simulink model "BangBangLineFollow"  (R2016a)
settings: Solver=FixedStepAuto  StartTime=0.0  StopTime=inf  RelTol=1e-3
libraries: miniQ x2

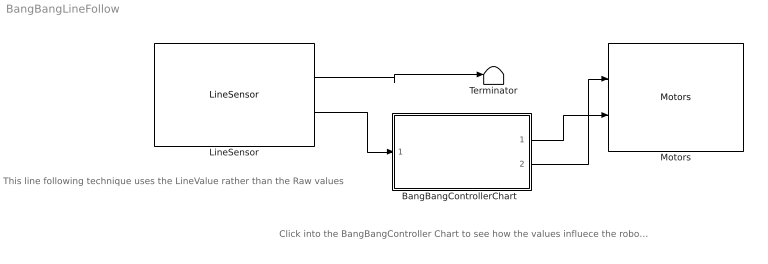
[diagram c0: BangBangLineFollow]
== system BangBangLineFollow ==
  note: Click into the BangBangController Chart to see how the values influece the robot's movement
  note: This line following technique uses the LineValue rather than the Raw values
  "BangBangControllerChart " : Stateflow chart  TreatAsAtomicUnit=on
  LineSensor : miniQ/LineSensor  sampleTime_dd=0.01  maxRawSensors=[800,900,900,900,800]  minRawSensors=[200,280,300,300,220]  debug_dd=off
  Motors : miniQ/Motors  flipLeft=off  flipRight=off
  Terminator : Terminator
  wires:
  LineSensor/2 -> "BangBangControllerChart "/1(value)
  "BangBangControllerChart "/1(r) -> Motors/2
  "BangBangControllerChart "/2(l) -> Motors/1
  LineSensor/1 -> Terminator/1

== stateflow chart BangBangLineFollow/BangBangControllerChart

 ==
  state Depending on if the robot is on the line or slightly to the inside of it the robot turns right or left [group]
    to hug the edge of the black line.
  state Forward
    entry: l=255
    r=255
  state Right
    entry: l=-150
    r=150
  state Left
    entry: l=150
    r=-150
  (default) -> Forward
  Left -> Forward : [value>2.90]
  Right -> Forward : [value<3.10]
  Forward -> Left : [value<2.90]
  Forward -> Right : [value>3.10]
  data: value input; r output; l output
